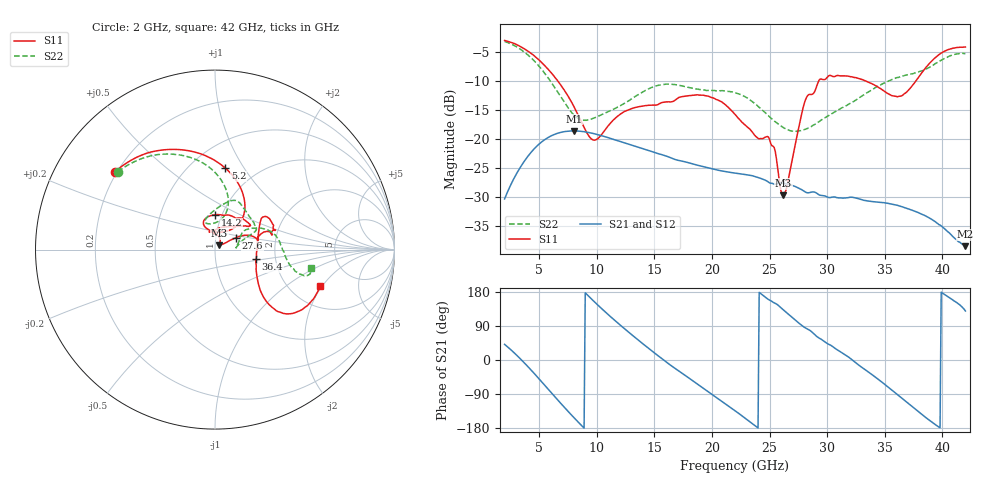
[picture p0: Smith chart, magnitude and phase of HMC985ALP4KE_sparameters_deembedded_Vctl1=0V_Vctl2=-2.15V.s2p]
!s2p File: Measurements: S11, S21, S12, S22
# GHz S dB R 50.0
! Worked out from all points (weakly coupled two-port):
!   401 points, 2 GHz to 42 GHz, reference 50 ohm
!   highest |S21| = -18.57 dB at 8 GHz (marker M1); lowest = -38.4 dB at 42 GHz (marker M2)
!   lowest |S11| = -29.7 dB at 26.2 GHz (marker M3), VSWR 1.07, Z = 52.3 + j2.42 ohm
!   |S11| at or under -10 dB: 6.623 GHz to 29.27 GHz (22.64 GHz wide, 126 % of centre); 33.37 GHz to 37.7 GHz (4.331 GHz wide, 12.2 % of centre)
!   |S22| runs from -18.7 to -3.2 dB; largest |S21 - S12| = 0.0004
!   S11 on the Smith chart (normalised r, x): 2 GHz: 0.19, +0.33; 5.2 GHz: 0.72, +0.83; 14.2 GHz: 0.93, +0.37; 27.6 GHz: 1.25, +0.17; 36.4 GHz: 1.58, -0.18; 42 GHz: 2.90, -1.91
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2  -3.02 142.4  -30.27 41.3  -30.27 41.3  -3.19 141.3
3.6  -4.32 113.3  -24.11 -4.0  -24.12 -4.1  -4.86 112.1
5.2  -6.78 82.9  -20.49 -56.9  -20.50 -56.9  -7.95 86.2
8  -14.32 47.4  -18.57 -151.5  -18.55 -151.5  -15.80 81.6
8.7  -17.18 52.3  -18.66 -173.6  -18.65 -173.6  -16.70 93.5
9.9  -20.12 88.9  -19.12 150.5  -19.13 150.5  -16.24 108.2
12.1  -15.61 112.9  -20.43 90.5  -20.46 90.4  -14.17 99.6
14.2  -14.23 89.8  -21.75 38.0  -21.73 38.0  -11.63 78.5
15.4  -13.94 73.2  -22.53 9.6  -22.50 9.6  -10.71 70.2
19.3  -12.45 34.2  -24.75 -75.3  -24.79 -75.4  -11.53 41.7
22  -15.71 52.3  -25.81 -133.7  -25.77 -133.7  -12.00 24.9
25  -20.04 98.6  -27.51 158.1  -27.55 158.0  -16.16 17.3
26.2  -29.68 44.7  -27.56 132.2  -27.61 132.1  -18.00 8.9
27.6  -17.38 29.7  -28.49 96.0  -28.49 96.0  -18.53 5.7
28.1  -13.31 20.9  -29.07 84.9  -29.06 84.8  -18.30 8.2
28.7  -12.28 13.0  -29.08 73.2  -29.04 73.3  -17.71 13.0
31  -9.06 23.3  -30.09 24.6  -30.09 24.5  -14.90 32.1
33.3  -9.94 34.2  -30.54 -25.5  -30.59 -25.5  -12.24 29.0
35.4  -12.27 12.1  -31.08 -74.2  -31.07 -74.2  -9.95 19.5
36.4  -12.58 -13.1  -31.56 -98.7  -31.53 -98.8  -9.19 13.4
39.5  -5.81 -43.4  -34.38 -172.9  -34.37 -172.8  -6.87 -13.9
42  -4.14 -19.0  -38.39 129.3  -38.45 129.4  -5.25 -10.9
